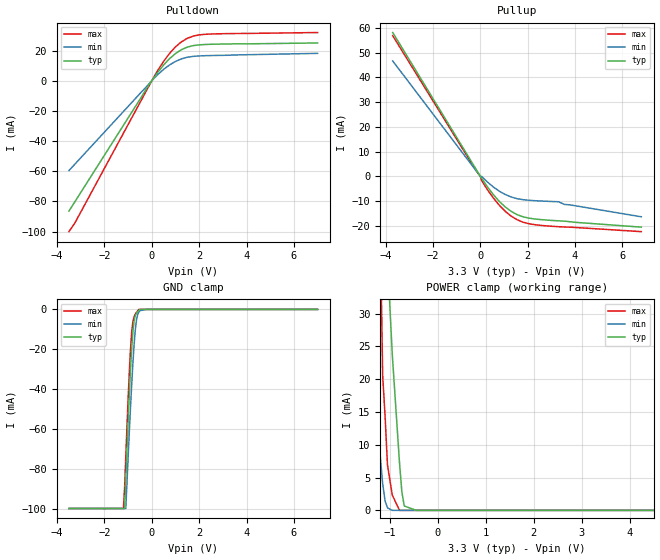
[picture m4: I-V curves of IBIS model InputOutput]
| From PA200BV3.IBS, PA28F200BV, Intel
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|********************Input Output Model**************************
[Model]   InputOutput
Model_type   I/O
|   Model for DQ[15:0] pins.
Vinl = 0.8V
Vinh = 2.0V
|Variable   Typ   Min   Max
C_comp   8.91p   NA   10.5p
[Voltage Range]   3.3V   3.0V   3.6V
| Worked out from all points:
|   slope of the pulldown table from 0 to 0.495 V, typ, clamps not added: 47.9 ohm
|   slope of the pullup table from 0 to 0.495 V, typ, clamps not added: 73.6 ohm
|   GND clamp passes 1 mA (typ) near -0.59 V on its own axis
|   POWER clamp passes 1 mA (typ) near -0.71 V on its own axis
[Pulldown]
| [Pullup] and [Pulldown] IV curves include only the current through
| the channels of output driver transistors when outputs are enabled
| with OE# = VIL.  Although the output driver transistors have np and
| pn diodes inherently created by CMOS IC fabrication between the
| drain and bulk of n-channel and p-channel CMOS transistors,
| the current through these junction diodes is not included in
| [Pullup] or [Pulldown].  Instead that drain/bulk diode current is
| included in the [POWER_clamp] or [GND_clamp] sections, which are
| not dependent on the state of OE# or output data value.
|Voltage   I(typ)   I(min)   I(max)
-3.5V     -86.38mA   -59.54mA   -100mA
-3.25V    -80.21mA   -55.29mA   -94.26mA
0V        0A         0A         0A
500mV     10.43mA    7.529mA    12.84mA
750mV     14.63mA    10.45mA    18.1mA
1V        18mA       12.77mA    22.41mA
1.25V     20.54mA    14.46mA    25.73mA
1.5V      22.25mA    15.55mA    28.08mA
1.75V     23.24mA    16.12mA    29.56mA
2.25V     23.98mA    16.55mA    30.72mA
7V        25mA       18.1mA     31.9mA
[GND_clamp]
| [POWER_clamp] and [GND_clamp] IV curves describe ESD protection
| circuits PLUS some np and pn diodes which exist between the
| drain and bulk of n-channel and p-channel CMOS transistors.
| These drain/bulk diodes are inherent in CMOS IC fabrication,
| and are visible on the node of the I/O pin at all times.
| Even the drain/bulk diodes of output driver [Pullup] and [Powerdown]
| transistors are included in [POWER_clamp] or [GND_clamp], because
| these diodes contribute to I/O pin current even when the
| chip outputs are tristated by OE# = VIH.
| For example, when V forced on the I/O pin is large, we are
| forward biasing the pn diode at the drain/bulk interface in the
| p-channel pullup transistor.  Similarly, when V forced on the
| I/O pin is sufficiently negative with respect to the substrate
| ground, we are forward biasing the np diode at the drain/bulk
| interface in the n-channel pulldown transistor.  The effects
| of these diodes are included in [POWER_clamp] or [GND_clamp].
|Voltage   I(typ)   I(min)   I(max)
-3.5V     -100mA     -100mA     -100mA
-1.2V     -100mA     -100mA     -100mA
-1.15V    -100mA     -100mA     -89.6mA
-1.1V     -85.3mA    -100mA     -74.13mA
-950mV    -42.6mA    -61.31mA   -31.32mA
-900mV    -30.13mA   -49.09mA   -19.82mA
-850mV    -19.6mA    -37.77mA   -11.26mA
-800mV    -11.17mA   -27.17mA   -6.11mA
-700mV    -3.17mA    -10.64mA   -2.365mA
-650mV    -1.862mA   -5.595mA   -1.442mA
-550mV    -543.9uA   -1.326mA   0A
7V        0A         0A         0A
[Pullup]
| (Voltages for [Pullup] and [POWER_clamp] are specified with
| negative respect to Vcc.  Reference the IBIS documentation
| for more information regarding Vtable = Vcc - Voutput.
| This method keeps -Vds constant for the values in all three
| columns across a line of the table.
| [Pullup] and [Pulldown] IV curves include only the current through
| the channels of output driver transistors when outputs are enabled
| with OE# = VIL.  Although the output driver transistors have np and
| pn diodes inherently created by CMOS IC fabrication between the
| drain and bulk of n-channel and p-channel CMOS transistors,
| the current through these junction diodes is not included in
| [Pullup] or [Pulldown].  Instead that drain/bulk diode current is
| included in the [POWER_clamp] or [GND_clamp] sections, which are
| not dependent on the state of OE# or output data value.
|Voltage  I(typ)   I(min)   I(max)
-3.7V     58.11mA    46.62mA    56.85mA
-200mV    3.163mA    2.529mA    2.54mA
0V        0A         0A         0A
50mV      -745.9uA   -11.29uA   -1.621mA
550mV     -7.415mA   -4.333mA   -8.771mA
1.05V     -12.38mA   -7.358mA   -14.14mA
1.3V      -14.17mA   -8.351mA   -16.1mA
1.8V      -16.37mA   -9.449mA   -18.55mA
2.3V      -17.27mA   -9.872mA   -19.57mA
3.3V      -18.01mA   -10.29mA   -20.38mA
3.55V     -18.14mA   -11.37mA   -20.51mA
6.8V      -20.56mA   -16.38mA   -22.38mA
[POWER_clamp]
| (Voltages for [Pullup] and [POWER_clamp] are specified with
| negative respect to Vcc.  Reference the IBIS documentation
| for more information regarding Vtable = Vcc - Voutput.
| This method keeps -Vds constant for the values in all three
| columns across a line of the table.
| [POWER_clamp] and [GND_clamp] IV curves describe ESD protection
| circuits PLUS some np and pn diodes which exist between the
| drain and bulk of n-channel and p-channel CMOS transistors.
| These drain/bulk diodes are inherent in CMOS IC fabrication,
| and are visible on the node of the I/O pin at all times.
| Even the drain/bulk diodes of output driver [Pullup] and [Powerdown]
| transistors are included in [POWER_clamp] or [GND_clamp], because
| these diodes contribute to I/O pin current even when the
| chip outputs are tristated by OE# = VIH.
| For example, when V forced on the I/O pin is large, we are
| forward biasing the pn diode at the drain/bulk interface in the
| p-channel pullup transistor.  Similarly, when V forced on the
| I/O pin is sufficiently negative with respect to the substrate
| ground, we are forward biasing the np diode at the drain/bulk
| interface in the n-channel pulldown transistor.  The effects
| of these diodes are included in [POWER_clamp] or [GND_clamp].
|Voltage I(typ)   I(min)   I(max)
-3.7V     100mA      100mA      100mA
-1.4V     94.2mA     32.79mA    74.44mA
-1.2V     63.86mA    8.261mA    43.03mA
-1.15V    56.35mA    4.04mA     20.56mA
-1.1V     48.95mA    1.449mA    14.38mA
-1.05V    38.43mA    383.6uA    6.922mA
-950mV    23.79mA    0A         2.34mA
-800mV    7.337mA    0A         0A
-750mV    2.782mA    0A         0A
-700mV    667.1uA    0A         0A
-450mV    0A         0A         0A
6.8V      0A         0A         0A
[Ramp]
| The DQ Ramp information is not provided at this time for the
| device but will be available in the future.  The table below
| is for the compatibility with some IBIS parsers.
| Variable   typ   min   max
 dV/dt_r   0V/0ns   0V/0ns   0V/0ns
 dV/dt_f   0V/0ns   0V/0ns   0V/0ns
